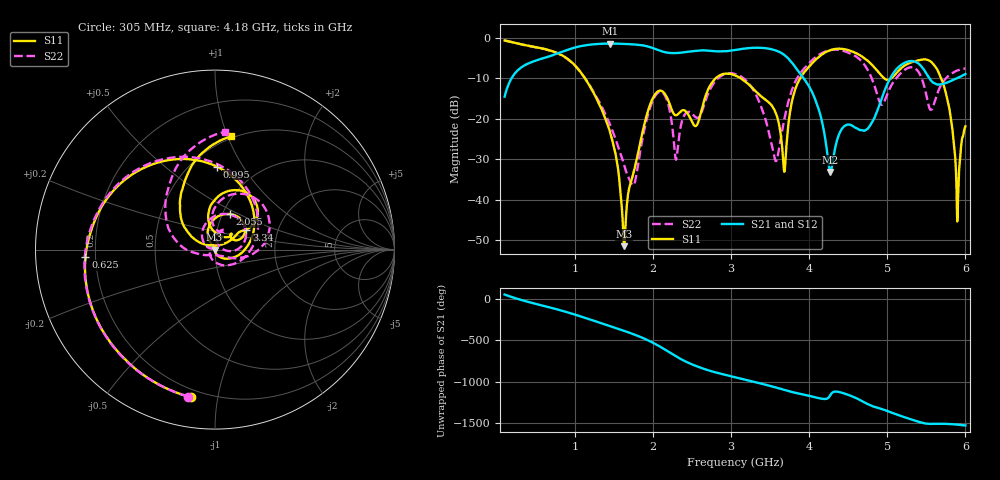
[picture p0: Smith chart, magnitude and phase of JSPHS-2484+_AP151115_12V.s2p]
!Mini-Circuits Laboratory
!S-Parameters
!Run/Lot/Date Code:MF33450/NA/1551
!Fixture/SN/Due: 90-4-20-21/70546/03/17/16
!Connection:PORT<IN> - pin<1>; PORT<OUT> - pin<7>;PORT<BIAS> - pin<4>;
!Tested With:PORT EXTENTION
!Network Analyzer:AG E5071C/74883/05/12/16
!Created: 01-07-2016 at 14:10:57
!MODEL: JSPHS-2484+
!S/N: V=12V
# MHZ S DB R 50
!Frequency  S11 dB  S11 DEG  S21 dB  S21 DEG  S12 dB  S12 DEG  S22 dB  S22 DEG
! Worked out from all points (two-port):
!   1181 points, 100 MHz to 6 GHz, reference 50 ohm
!   highest |S21| = -1.44 dB at 1.455 GHz (marker M1); lowest = -33.1 dB at 4.27 GHz (marker M2)
!   |S21| within 3 dB of the highest: 696 MHz to 3.694 GHz (2.998 GHz wide, 137 % of centre)
!   lowest |S11| = -51.4 dB at 1.63 GHz (marker M3), VSWR 1.01, Z = 49.7 - j0.034 ohm
!   |S11| at or under -10 dB: 1.129 GHz to 2.802 GHz (1.674 GHz wide, 85.2 % of centre); 3.124 GHz to 3.886 GHz (761.5 MHz wide, 21.7 % of centre); 5.69 GHz to end of sweep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
!   |S22| runs from -36.4 to -0.7 dB; largest |S21 - S12| = 0.0042
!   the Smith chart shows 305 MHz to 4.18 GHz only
!   S11 on the Smith chart (normalised r, x): 305 MHz: 0.16, -0.84; 625 MHz: 0.16, -0.03; 995 MHz: 0.66, +0.78; 2.055 GHz: 1.09, +0.45; 3.34 GHz: 1.38, +0.32; 4.18 GHz: 0.48, +1.03
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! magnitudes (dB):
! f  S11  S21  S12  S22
! 100 MHz  -0.7  -14.5  -14.5  -0.7
! 305 MHz  -1.6  -7.4  -7.4  -1.6
! 625 MHz  -2.8  -4.9  -4.9  -2.9
! 995 MHz  -6.7  -2.4  -2.4  -6.8
! 1.085 GHz  -8.8  -2.0  -2.0  -8.8
! 1.455 GHz  -23.6  -1.4  -1.4  -21.7
! 1.63 GHz  -51.4  -1.5  -1.5  -31.3
! 1.76 GHz  -32.6  -1.7  -1.6  -36.1
! 2.055 GHz  -13.4  -2.9  -2.9  -13.7
! 2.07 GHz  -13.2  -3.1  -3.1  -13.5
! 2.295 GHz  -19.1  -3.8  -3.8  -30.1
! 3.05 GHz  -9.3  -3.0  -3.0  -8.9
! 3.34 GHz  -13.7  -2.5  -2.5  -14.9
! 3.57 GHz  -18.4  -3.1  -3.1  -30.4
! 3.68 GHz  -33.1  -4.2  -4.2  -20.3
! 4.035 GHz  -6.3  -13.3  -13.3  -5.6
! 4.18 GHz  -3.9  -22.2  -22.3  -3.6
! 4.27 GHz  -3.1  -33.1  -32.9  -3.0
! 5.02 GHz  -10.3  -10.6  -10.6  -13.0
! 5.625 GHz  -7.4  -11.4  -11.4  -14.6
! 5.9 GHz  -44.2  -9.9  -9.9  -8.1
! 6 GHz  -21.9  -8.9  -9.0  -7.6
